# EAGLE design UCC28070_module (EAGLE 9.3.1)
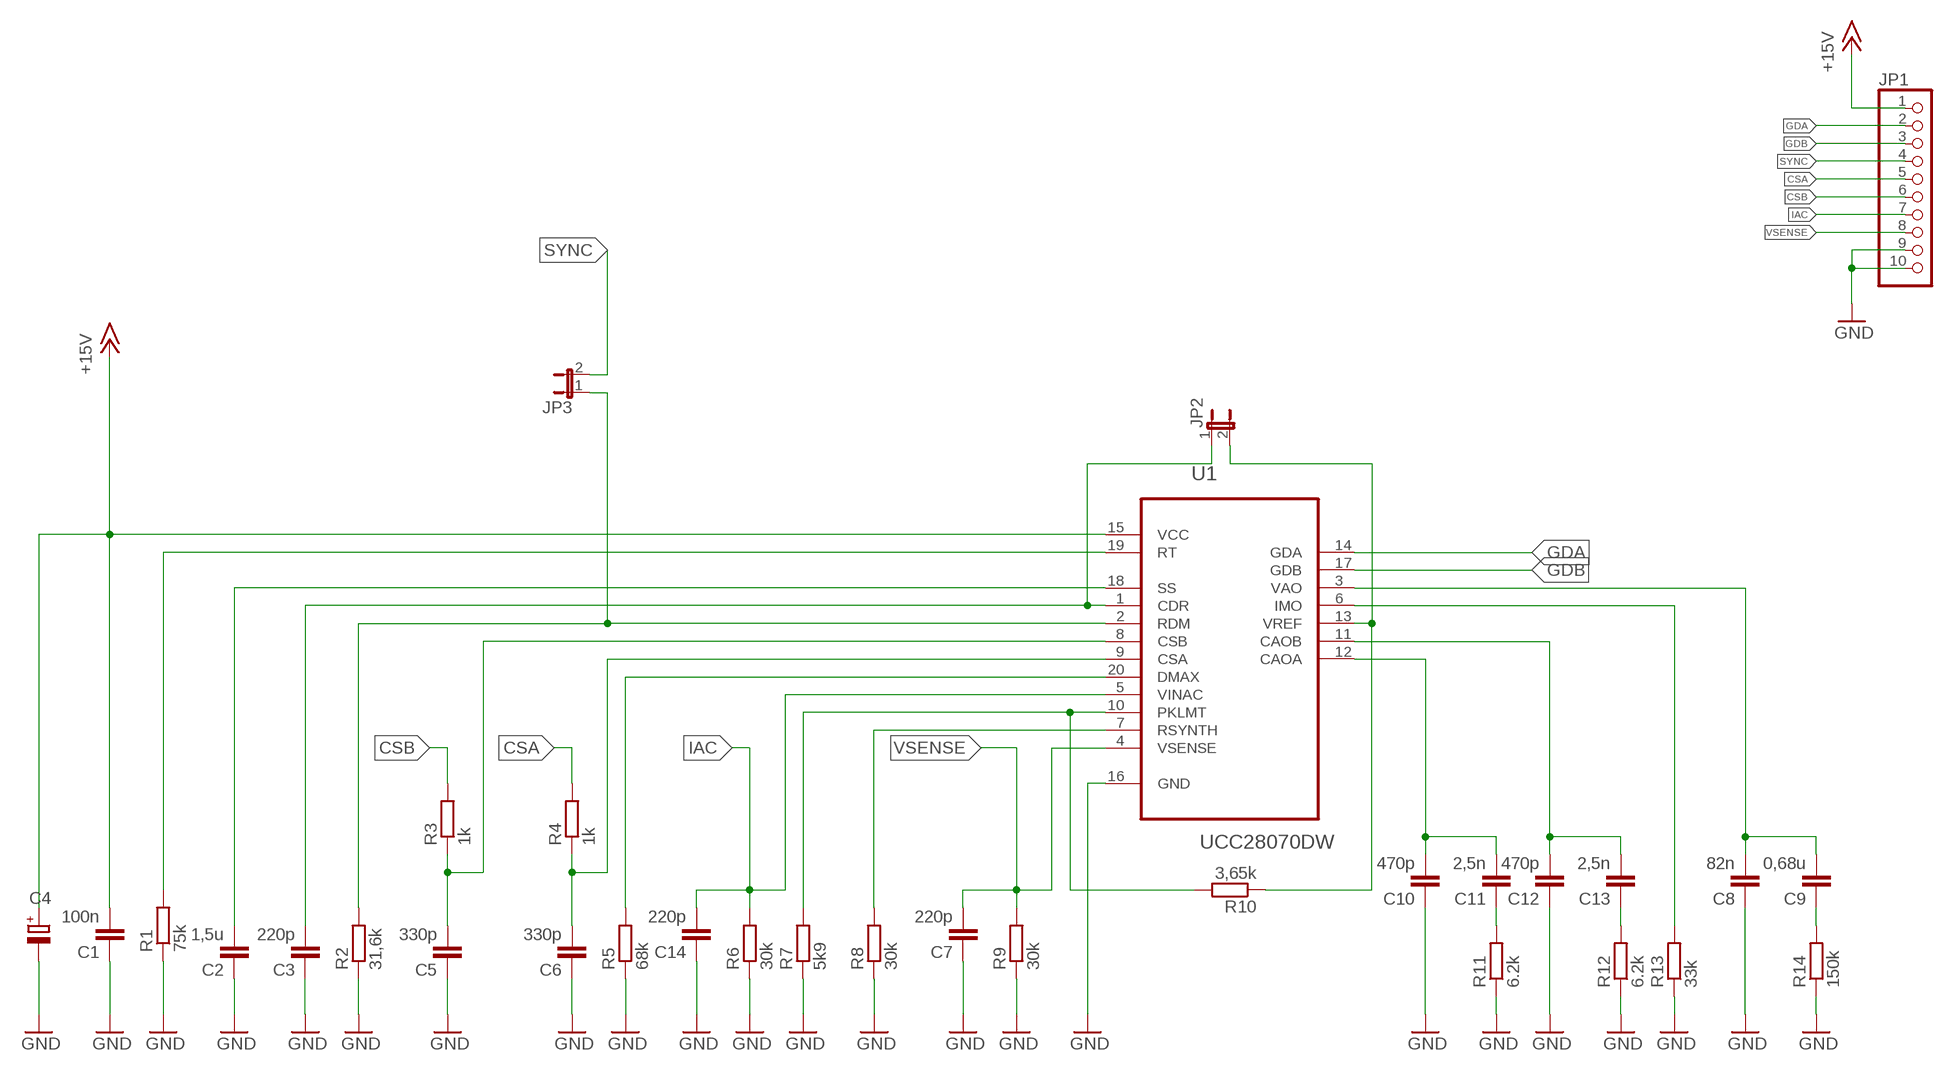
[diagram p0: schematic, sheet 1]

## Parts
C1  100n  C-EU0805  [0805_HT]
C2  1,5u  C-EU0805  [0805_HT]
C3  220p  C-EU0805  [0805_HT]
C4  CPOL-EUE2.5-7  [E2,5-7]
C5  330p  C-EU0805  [0805_HT]
C6  330p  C-EU0805  [0805_HT]
C7  220p  C-EU0805  [0805_HT]
C8  82n  C-EU0805  [0805_HT]
C9  0,68u  C-EU0805  [0805_HT]
C10  470p  C-EU0805  [0805_HT]
C11  2,5n  C-EU0805  [0805_HT]
C12  470p  C-EU0805  [0805_HT]
C13  2,5n  C-EU0805  [0805_HT]
C14  220p  C-EU0805  [0805_HT]
JP1  PINHD-1X10/90  [1X10/90]
JP2  JP1E  [JP1]
JP3  JP1E  [JP1]
R1  75k  R-EU0805  [0805_HT]
R2  31,6k  R-EU0805  [0805_HT]
R3  1k  R-EU0805  [0805_HT]
R4  1k  R-EU0805  [0805_HT]
R5  68k  R-EU0805  [0805_HT]
R6  30k  R-EU0805  [0805_HT]
R7  5k9  R-EU0805  [0805_HT]
R8  30k  R-EU0805  [0805_HT]
R9  30k  R-EU0805  [0805_HT]
R10  3,65k  R-EU0805  [0805_HT]
R11  6.2k  R-EU0805  [0805_HT]
R12  6.2k  R-EU0805  [0805_HT]
R13  33k  R-EU0805  [0805_HT]
R14  150k  R-EU0805  [0805_HT]
U1  UCC28070DW  [SOIC127P1030X265-20N]

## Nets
+15V: C1.2 C4.+ JP1.1 U1.15(VCC)
CSA: JP1.5 R4.2
CSB: JP1.6 R3.2
GDA: JP1.2 U1.14(GDA)
GDB: JP1.3 U1.17(GDB)
GND: C1.1 C2.1 C3.1 C4.- C5.1 C6.1 C7.1 C8.1 C10.1 C12.1 C14.1 JP1.9 JP1.10 R1.1 R2.1 R5.1 R6.1 R7.1 R8.1 R9.1 R11.1 R12.1 R13.1 R14.1 U1.16(GND)
IAC: C14.2 JP1.7 R6.2 U1.5(VINAC)
N$37: R1.2 U1.19(RT)
N$38: C3.2 JP2.1 U1.1(CDR)
N$40: R8.2 U1.7(RSYNTH)
N$41: R7.2 R10.2 U1.10(PKLMT)
N$42: JP2.2 R10.1 U1.13(VREF)
N$43: R13.2 U1.6(IMO)
N$44: C8.2 C9.2 U1.3(VAO)
N$45: C11.1 R11.2
N$46: C10.2 C11.2 U1.12(CAOA)
N$47: C12.2 C13.2 U1.11(CAOB)
N$48: C13.1 R12.2
N$49: C9.1 R14.2
N$51: R5.2 U1.20(DMAX)
N$52: C6.2 R4.1 U1.9(CSA)
N$53: C5.2 R3.1 U1.8(CSB)
N$54: JP3.1 R2.2 U1.2(RDM)
N$55: C2.2 U1.18(SS)
SYNC: JP1.4 JP3.2
VSENSE: C7.2 JP1.8 R9.2 U1.4(VSENSE)

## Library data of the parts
C1-C3 C5-C14 = HT_components:C-EU
C4 = rcl:CPOL-EU: POLARIZED CAPACITOR, European symbol; SPICEPREFIX: C
JP1 = pinhead:PINHD-1X10: PIN HEADER
JP2 JP3 = jumper:JP1E: JUMPER
R1-R14 = HT_components:R-EU
U1 = Texas Instruments_By_element14_Batch_1:UCC28070DW: Interleaving Continuous Conduction Mode PFC Controller; MPN: UCC28070DW; OC_FARNELL: -; OC_NEWARK: 25R0172; PACKAGE: SOIC-20; SUPPLIER: Texas Instruments

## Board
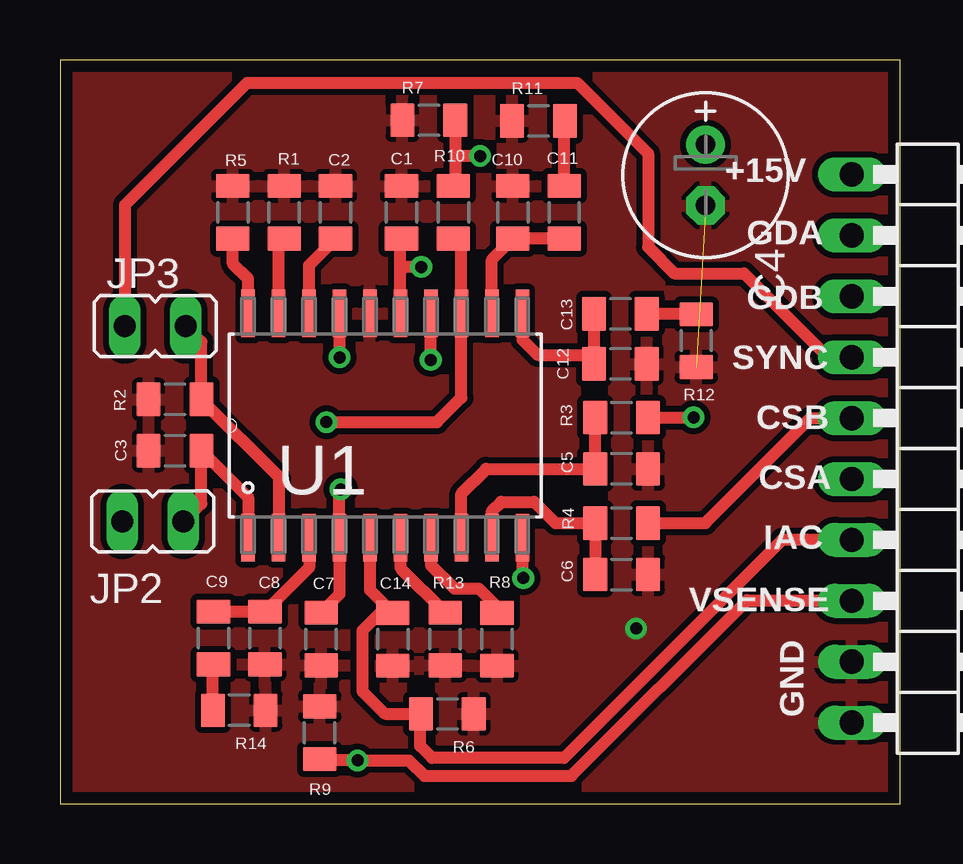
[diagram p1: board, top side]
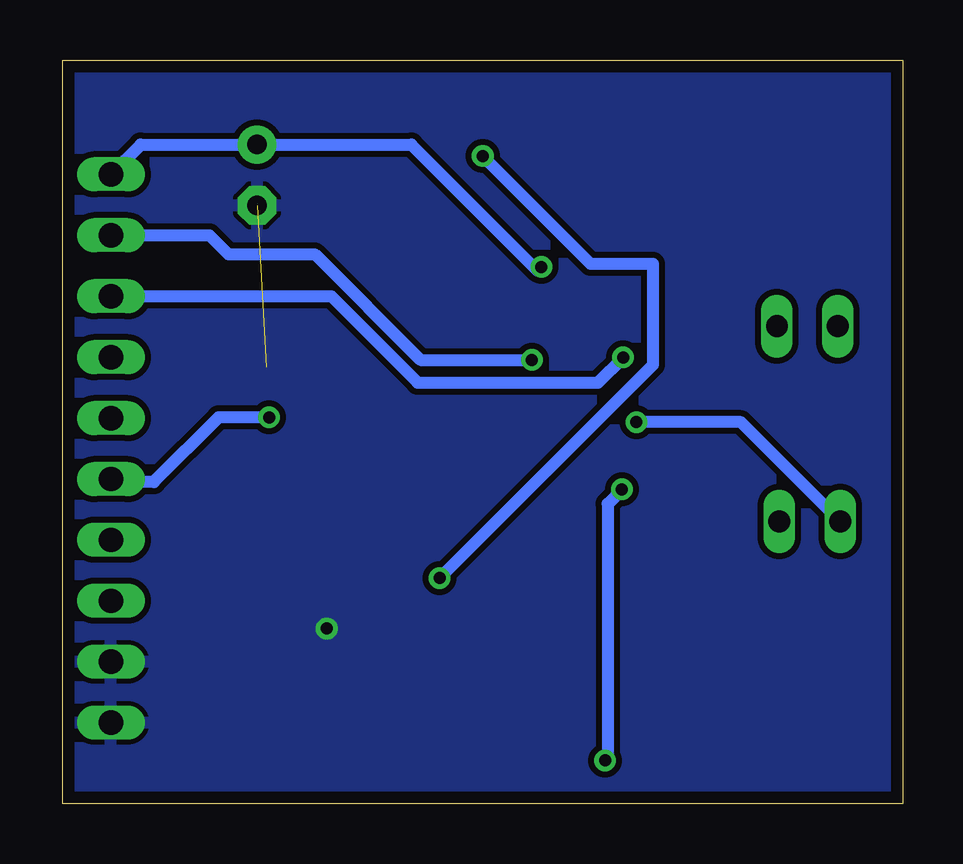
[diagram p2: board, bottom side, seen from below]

Size 35 x 31 mm. Coordinates in mm from the lower left corner, seen from the top.
Outline: 0,0 35,0 35,31 0,31 0,0
Copper layers (1*16): Top 0.035mm / dielectric 1.5mm / Bottom 0.035mm
Design rules "EVC_stadard": minimum track width 0.5mm, minimum drill 0.5mm, track to track 0.25mm, track to pad 0.25mm, pad to pad 0.5mm, via to via 0.5mm, smd to smd 0.15mm, copper to edge 0.5mm, drill to drill 0.5mm, minimum pad ring 0.2mm, minimum via ring 0.2mm, stop-mask expansion 0.075mm, vias tented up to drill 0mil, thermal gap 0.2mm

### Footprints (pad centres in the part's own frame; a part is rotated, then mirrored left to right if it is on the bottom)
0805_HT = smd 1 x 1.4: 1 -1.1,0; 2 1.1,0
E2,5-7 = drill 0.813 pad 1.6: + -1.27,0 | drill 0.813 pad 1.6 octagon: - 1.27,0
1X10/90 = drill 1.016 long: 1 -11.43,-3.81; 2 -8.89,-3.81; 3 -6.35,-3.81; 4 -3.81,-3.81; 5 -1.27,-3.81; 6 1.27,-3.81; 7 3.81,-3.81; 8 6.35,-3.81; 9 8.89,-3.81; 10 11.43,-3.81
JP1 = drill 0.914 long: 1 0,-1.27; 2 0,1.27
SOIC127P1030X265-20N = smd 1.981 x 0.559: 1 -4.674,5.715; 2 -4.674,4.445; 3 -4.674,3.175; 4 -4.674,1.905; 5 -4.674,0.635; 6 -4.674,-0.635; 7 -4.674,-1.905; 8 -4.674,-3.175; 9 -4.674,-4.445; 10 -4.674,-5.715; 11 4.674,-5.715; 12 4.674,-4.445; 13 4.674,-3.175; 14 4.674,-1.905; 15 4.674,-0.635; 16 4.674,0.635; 17 4.674,1.905; 18 4.674,3.175; 19 4.674,4.445; 20 4.674,5.715

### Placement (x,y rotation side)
C1  14.23,24.65 270 top
C2  11.48,24.65 270 top
C3  4.79,14.71 0 top
C4  26.9,26.2 270 top
C5  23.4,13.95 180 top
C6  23.4,9.55 180 top
C7  10.88,6.86 90 top
C8  8.54,6.9 90 top
C9  6.4,6.9 90 top
C10  18.87,24.65 270 top
C11  21.01,24.65 270 top
C12  23.35,18.33 180 top
C13  23.35,20.42 180 top
C14  13.87,6.85 90 top
JP1  36.8,14.8 270 top
JP2  3.87,11.76 90 top
JP3  3.97,19.9 90 top
R1  9.34,24.65 270 top
R2  4.79,16.85 0 top
R3  23.4,16.09 0 top
R4  23.4,11.69 0 top
R5  7.2,24.65 270 top
R6  16.14,3.74 180 top
R7  15.37,28.49 0 top
R8  18.21,6.85 90 top
R9  10.82,2.95 270 top
R10  16.39,24.65 90 top
R11  19.94,28.46 0 top
R12  26.51,19.3 90 top
R13  16.05,6.86 90 top
R14  7.47,3.89 180 top
U1  13.55,15.76 90 top

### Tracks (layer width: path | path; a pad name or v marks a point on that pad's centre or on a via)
+15V  (via drill 0.5)
  Top 0.5: U1.15 14.19,22.2 | 14.19,22.2 14.19,23.5 C1.2 | v15.05,22.37 14.36,22.37 14.19,22.2
  Bottom 0.5: v15.05,22.37 15.05,22.35 15.2,22.2 20.47,27.47 C4.+ 31.75,27.47 JP1.1
CSA
  Top 0.5: R4.2 26.89,11.69 31.27,16.07 JP1.5
CSB  (via drill 0.5)
  Top 0.5: 24.52,16.07 R3.2 v26.39,16.09 v26.4,16.1
  Bottom 0.5: v26.4,16.1 28.5,16.1 31.2,13.4 32.86,13.4 JP1.6
GDA  (via drill 0.5)
  Top 0.5: v15.45,18.5 U1.14
  Bottom 0.5: v15.45,18.5 20.1,18.5 24.5,22.9 28.1,22.9 28.89,23.69 JP1.2
GDB  (via drill 0.5)
  Top 0.5: v11.65,18.6 U1.17
  Bottom 0.5: JP1.3 23.81,21.15 20.21,17.55 12.7,17.55 v11.65,18.6
GND  (via drill 0.5)  (1 unrouted)
  other vias: 24,7.3
  pour Top: 0,0 35,0 35,31 0,31
  pour Bottom: 0,0 35,0 35,31 0,31
IAC
  Top 0.5: U1.5 12.91,8.9 C14.2 13.35,7.95 12.6,7.2 12.6,4.68 13.54,3.74 15,3.74 | 15,3.74 R6.2 | JP1.7 30.09,10.99 21,1.9 15.5,1.9 15,2.4 15,3.74
N$37
  Top 0.5: U1.19 9.11,23.32 R1.2
N$38
  Top 0.5: U1.1 7.83,12.77 C3.2 5.89,12.51 JP2.1
N$40
  Top 0.5: U1.7 15.46,9.95 16.44,8.96 17.44,8.96 18.21,8.19 R8.2
N$41  (via drill 0.5)
  Top 0.5: R7.2 16.47,27 | 16.47,27 16.47,25.83 R10.2 | v17.5,27 16.47,27 | U1.10 19.27,9.44 v19.3,9.4
  Bottom 0.5: v17.5,27 13,22.5 10.4,22.5 10.4,18.6 10.4,18.5 10.4,18.3 v19.3,9.4
N$42  (via drill 0.5)
  Top 0.5: R10.1 16.73,23.21 U1.13 16.73,16.93 15.7,15.9 v11.1,15.9
  Bottom 0.5: JP2.2 6.74,15.9 v11.1,15.9
N$43
  Top 0.5: U1.6 14.19,9.82 R13.2
N$44
  Top 0.5: U1.3 10.38,9.84 C8.2 C9.2
N$45
  Top 0.5: C11.1 21.01,28.43 R11.2
N$46
  Top 0.5: U1.12 18,22.68 C10.2 C11.2
N$47
  Top 0.5: C12.2 22.25,18.7 | 22.25,18.7 C13.2 | U1.11 19.27,19.34 19.9,18.7 22.25,18.7
N$48
  Top 0.5: C13.1 26.49,20.42 R12.2
N$49
  Top 0.5: R14.2 6.37,5.77 C9.1
N$51
  Top 0.5: U1.20 7.83,21.86 7.2,22.5 R5.2
N$52
  Top 0.5: U1.9 18,12.2 18.38,12.58 19.75,12.58 20.64,11.69 R4.1 C6.2
N$53
  Top 0.5: R3.1 C5.2 17.75,13.95 16.73,12.93 U1.8
N$54
  Top 0.5: U1.2 9.11,13.63 R2.2 5.89,19.25 JP3.1
N$55
  Top 0.5: U1.18 10.38,22.45 C2.2
SYNC
  Top 0.5: JP3.2 2.7,24.95 7.8,30.05 21.55,30.05 24.5,27.1 24.5,23.2 25.6,22.1 28.5,22.1 31.99,18.61 JP1.4
VSENSE  (via drill 0.5)
  Top 0.5: C7.2 11.64,8.72 U1.4 11.64,13.04 v11.7,13.1 | R9.2 10.87,1.8 v12.4,1.8 14.54,1.8 15.19,1.15 21.31,1.15 28.63,8.47 32.97,8.47 JP1.8
  Bottom 0.5: v12.4,1.8 12.3,1.8 12.3,12.5 v11.7,13.1

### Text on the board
tNames: +15V | GDA | GDB | SYNC | CSB | CSA | IAC | VSENSE | GND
